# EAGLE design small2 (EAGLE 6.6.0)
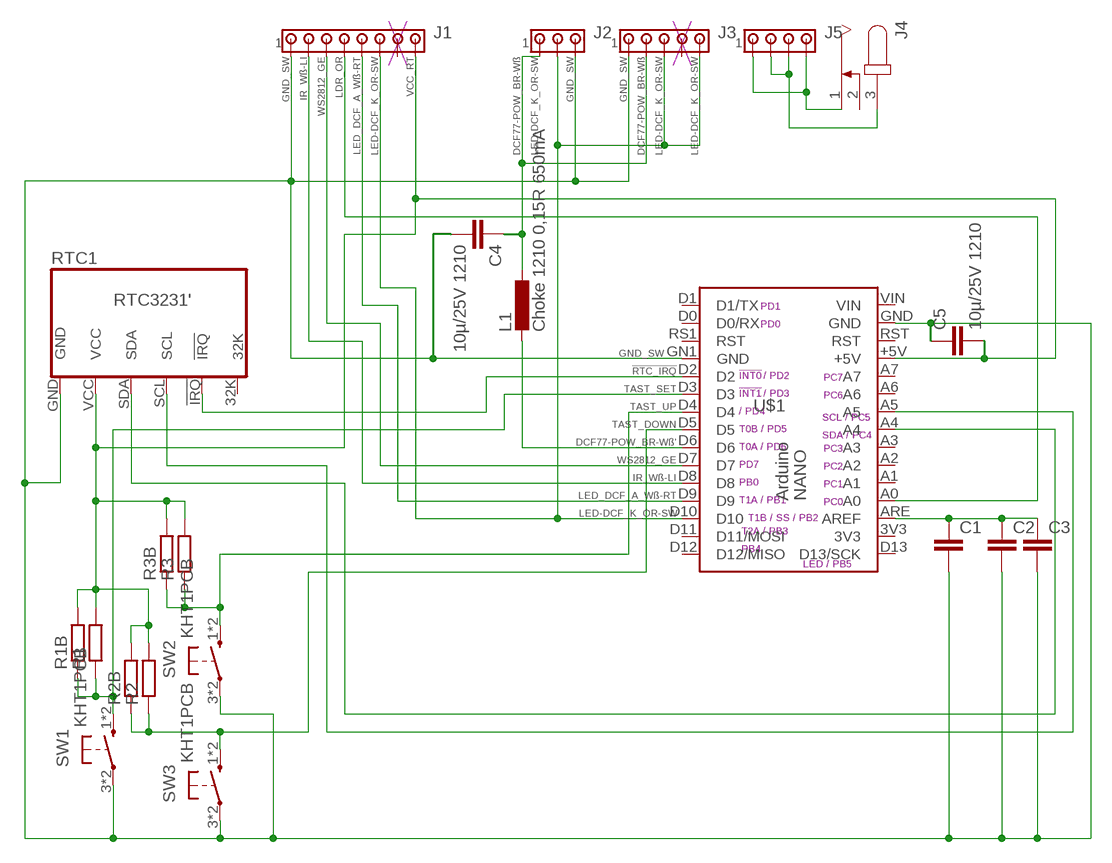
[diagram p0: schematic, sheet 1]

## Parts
C1  C-EU025-024X044  [C025-024X044]
C2  C-EU050-024X044  [C050-024X044]
C3  C-EUC0805  [C0805]
C4  10µ/25V 1210  C-EUC1210  [C1210]
C5  10µ/25V 1210  C-EUC1210  [C1210]
J1  MTA08-100  [10X08MTA]
J2  MTA03-100  [10X03MTA]
J3  MTA05-100  [10X05MTA]
J4  JACK-PLUG0  [SPC4077]
J5  MTA04-100  [10X04MTA]
L1  Choke 1210 0,15R 650mA  L-EUL2825P  [L2825P]
R1  R-EU_0204/5  [0204/5]
R1B  R-EU_M0805  [M0805]
R2  R-EU_0204/5  [0204/5]
R2B  R-EU_R0805  [R0805]
R3  R-EU_0204/5  [0204/5]
R3B  R-EU_M0805  [M0805]
RTC1  RTC3231'  [RTC3231"]
SW1  KHT1PCB  [OMRON_SWITCH]
SW2  KHT1PCB  [OMRON_SWITCH]
SW3  KHT1PCB  [OMRON_SWITCH]
U$1  ARDUINO_NANO3"  [ARDUINO_NANO3"]

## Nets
!RTC_IRQ: RTC1.!IRQ U$1.D2
DCF77-POW_BR-Wß: C4.1 J2.1 J3.2 L1.1
DCF77-POW_BR-Wß': L1.2 U$1.D6
GND_SW: C1.2 C2.2 C3.2 C4.2 C5.1 J1.1 J2.3 J3.1 RTC1.GND SW1.3(S) SW1.4(S) SW2.3(S) SW2.4(S) SW3.3(S) SW3.4(S) U$1.GN1(GND) U$1.GND
IR_Wß-LI: J1.2 U$1.D8
LDR_OR: J1.4 U$1.A0
LED-DCF_K_OR-SW: J1.6 J2.2 J3.3 J3.5 U$1.D10
LED_DCF_A_Wß-RT: J1.5 U$1.D9
N$2: RTC1.SDA U$1.A4
N$3: RTC1.SCL U$1.A5
N$6: C1.1 C2.1 C3.1 U$1.ARE(AREF)
N$78: J4.3 J5.2 J5.3
N$79: J4.1 J5.1 J5.4
TAST_DOWN: R2.1 R2B.1 SW3.1(P) SW3.2(P) U$1.D5
TAST_SET: R1.1 R1B.1 SW1.1(P) SW1.2(P) U$1.D3
TAST_UP: R3.1 R3B.1 SW2.1(P) SW2.2(P) U$1.D4
VCC_RT: C5.2 J1.8 R1.2 R1B.2 R2.2 R2B.2 R3.2 R3B.2 RTC1.VCC U$1.+5V
WS2812_GE: J1.3 U$1.D7
Unconnected: J1.7 J3.4 J4.2 RTC1.32K U$1.A1 U$1.A2 U$1.A3 U$1.A6 U$1.A7 U$1.D0(D0/RX) U$1.D1(D1/TX) U$1.D11(D11/MOSI) U$1.D12(D12/MISO) U$1.D13(D13/SCK) U$1.RS1(RST) U$1.RST

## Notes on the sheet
- GND_SW

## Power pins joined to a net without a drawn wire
3V3: U$1.3V3
VIN: U$1.VIN

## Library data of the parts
C1-C5 = rcl:C-EU: CAPACITOR, European symbol
J1 = con-amp:MTA08-100: AMP connector
J2 = con-amp:MTA03-100: AMP connector
J3 = con-amp:MTA05-100: AMP connector
J4 = con-jack:JACK-PLUG: DC POWER JACK Power Jack, DC, Right Angle, Through Hole, Rated 5A at 16VDC, PC Terminals Distributor: Farnell (www.Farnell.de) Drawing: 84N1161.pdf / 84N1162.pdf Manufacturer: SPC Technology (www.spctechnology.com) Type: SPC4077 / SPC 4078; OC_FARNELL: unknown; OC_NEWARK: unknown
J5 = con-amp:MTA04-100: AMP connector
L1 = rcl:L-EU: INDUCTOR, European symbol
R1 R1B R2 R2B R3 R3B = rcl:R-EU_: RESISTOR, European symbol
RTC1 = 1_____my_____1:RTC3231
SW1-SW3 = 1_____my_____1:KHT1
U$1 = 1_____my_____1:ARDUINO_NANO3

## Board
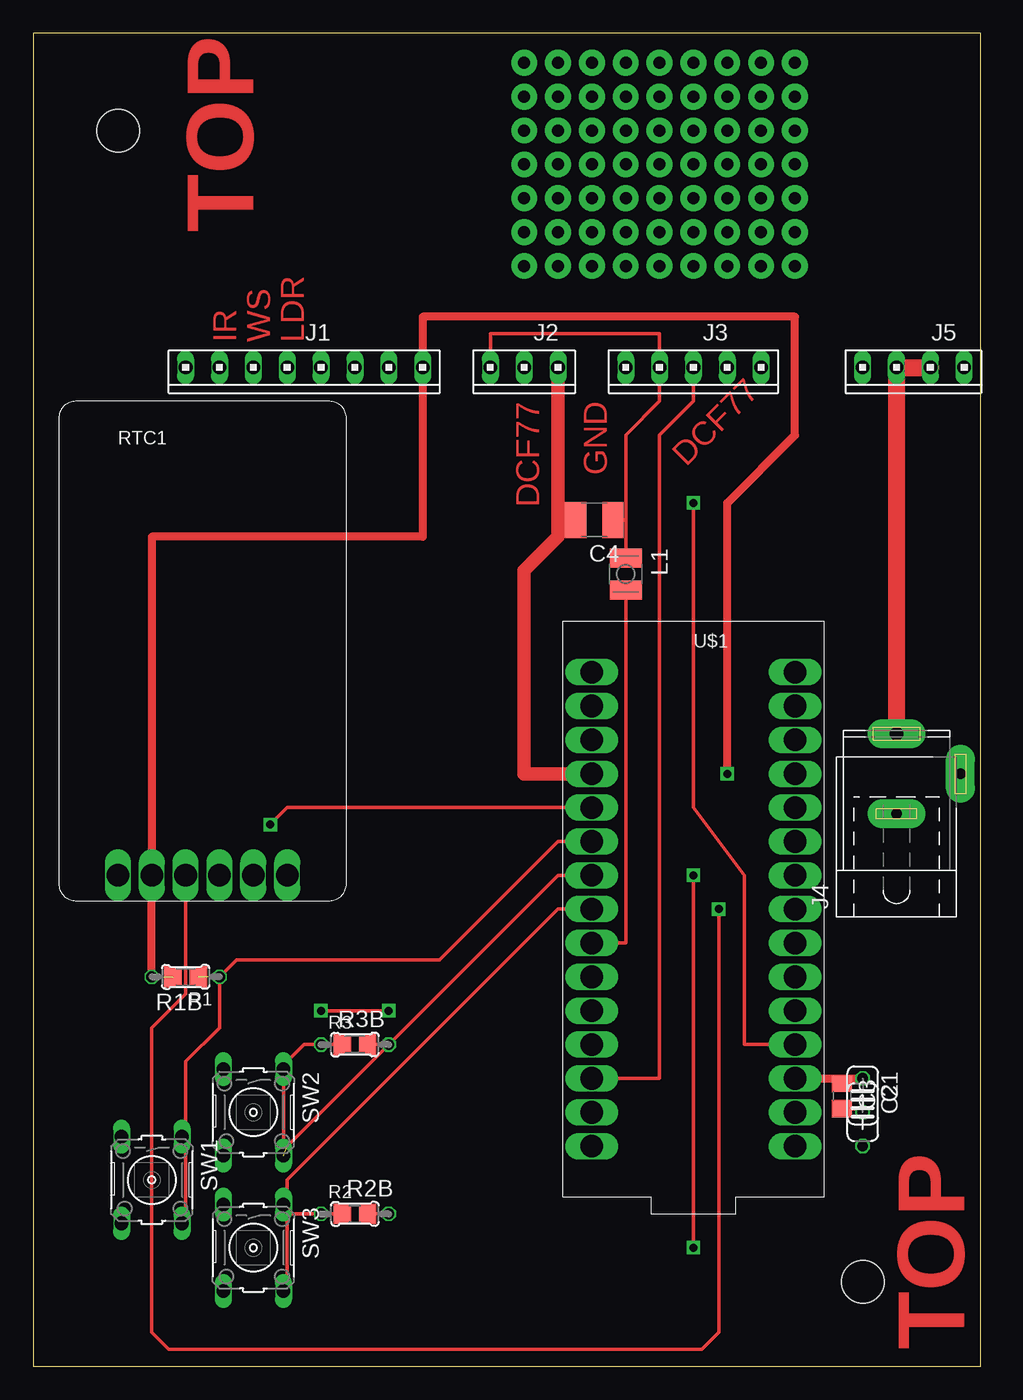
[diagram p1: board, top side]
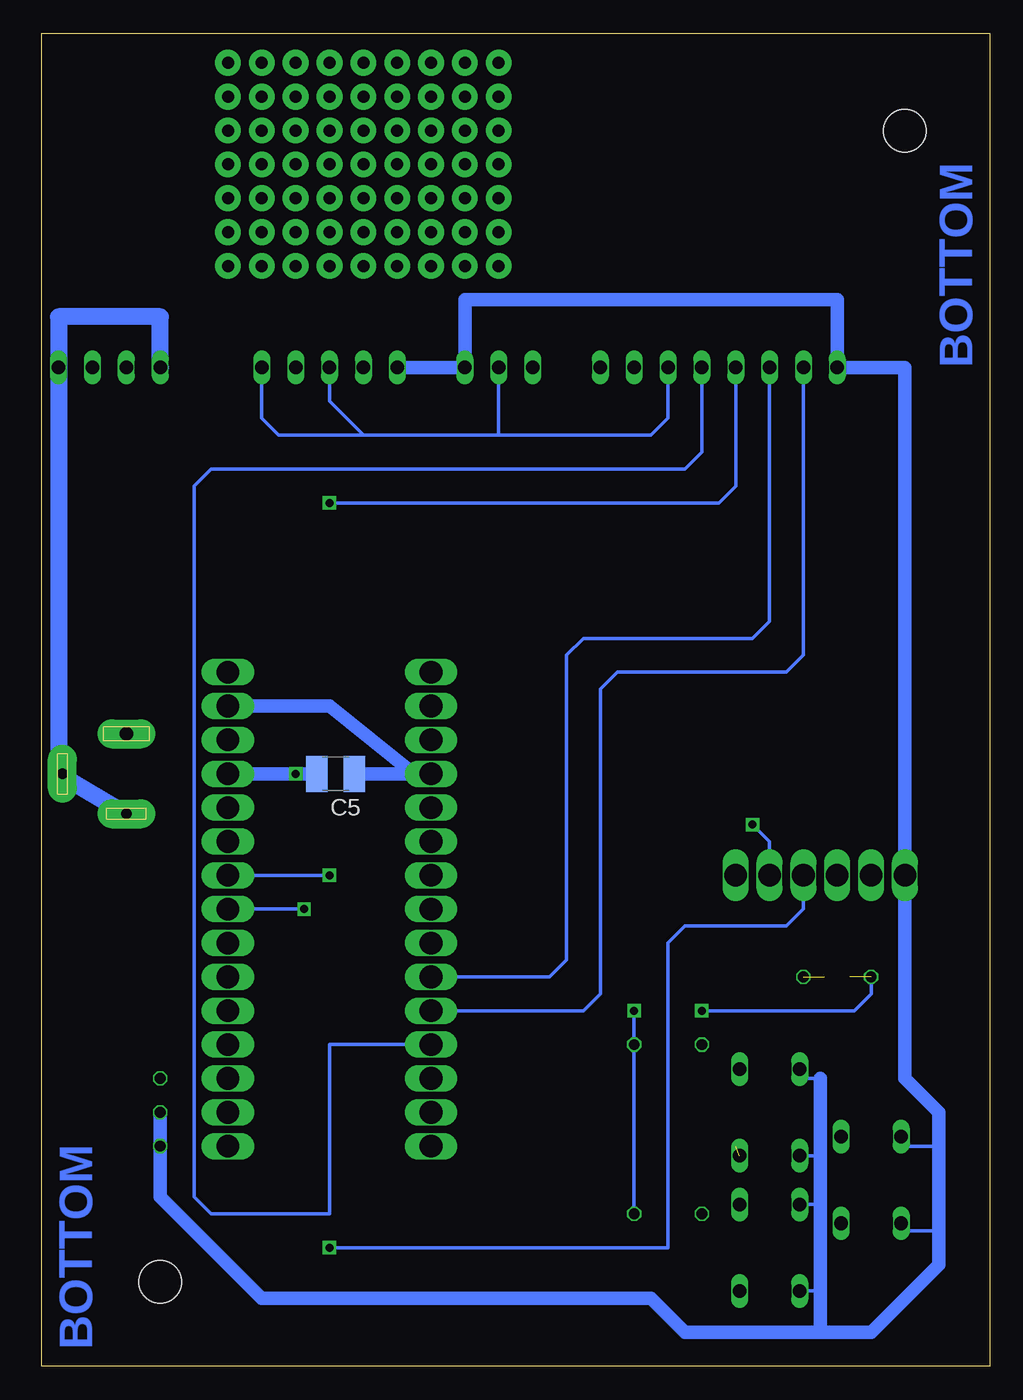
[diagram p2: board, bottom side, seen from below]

Size 71.11 x 100 mm. Coordinates in mm from the lower left corner, seen from the top.
Outline: 0,0 71.11,0 71.11,100 0,100 0,0
Copper layers (1*16): Top 0.035mm / dielectric 1.5mm / Bottom 0.035mm
Design rules "default *": minimum track width 10mil, minimum drill 24mil, track to track 8mil, track to pad 8mil, pad to pad 8mil, via to via 8mil, smd to smd 8mil, copper to edge 40mil, drill to drill 8mil, minimum pad ring 5mil, minimum via ring 8mil, stop-mask expansion 4mil, vias tented up to drill 0mil, thermal gap 10mil
Holes 3.2 mm at 6.35,92.71 62.23,6.35

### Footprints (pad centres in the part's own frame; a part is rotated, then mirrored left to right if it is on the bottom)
C025-024X044 = drill 0.813 octagon: 1 -1.27,0; 2 1.27,0
C050-024X044 = drill 0.813 octagon: 1 -2.54,0; 2 2.54,0
C0805 = smd 1.3 x 1.5: 1 -0.95,0; 2 0.95,0
C1210 = smd 1.6 x 2.7: 1 -1.4,0; 2 1.4,0
10X08MTA = drill 1.016 long: 1 8.89,0; 2 6.35,0; 3 3.81,0; 4 1.27,0; 5 -1.27,0; 6 -3.81,0; 7 -6.35,0; 8 -8.89,0
10X03MTA = drill 1.016 long: 1 2.54,0; 2 0,0; 3 -2.54,0
10X05MTA = drill 1.016 long: 1 5.08,0; 2 2.54,0; 3 0,0; 4 -2.54,0; 5 -5.08,0
SPC4077 = drill 0.8 pad 2.184 long: 1 -3,0; 2 0,-4.8 | drill 1 pad 2.184 long: 3 3,0
10X04MTA = drill 1.016 long: 1 3.81,0; 2 1.27,0; 3 -1.27,0; 4 -3.81,0
L2825P = smd 1.4 x 2.4: 1 -1.2,0; 2 1.2,0
0204/5 = drill 0.813 octagon: 1 -2.54,0; 2 2.54,0
M0805 = smd 1.3 x 1.6: 1 -0.95,0; 2 0.95,0
R0805 = smd 1.3 x 1.5: 1 -0.95,0; 2 0.95,0
RTC3231" = drill 1.7 pad 1.778 long: 32K 12.7,0; !IRQ 10.16,0; GND 0,0; SCL 7.62,0; SDA 5.08,0; VCC 2.54,0
OMRON_SWITCH = drill 1.016 long: 1 -3.251,2.261; 2 3.251,2.261; 3 -3.251,-2.261; 4 3.251,-2.261
ARDUINO_NANO3" = drill 1.7 pad 1.981 long: 3V3 15.24,-33.02; +5V 15.24,-7.62; A0 15.24,-27.94; A1 15.24,-25.4; A2 15.24,-22.86; A3 15.24,-20.32; A4 15.24,-17.78; A5 15.24,-15.24; A6 15.24,-12.7; A7 15.24,-10.16; ARE 15.24,-30.48; D0 0,-2.54; D1 0,0; D2 0,-10.16; D3 0,-12.7; D4 0,-15.24; D5 0,-17.78; D6 0,-20.32; D7 0,-22.86; D8 0,-25.4; D9 0,-27.94; D10 0,-30.48; D11 0,-33.02; D12 0,-35.56; D13 15.24,-35.56; GN1 0,-7.62; GND 15.24,-2.54; RS1 0,-5.08; RST 15.24,-5.08; VIN 15.24,0

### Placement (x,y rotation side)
C1  62.23,20.32 270 top
C2  62.23,19.05 270 top
C3  60.68,20.27 270 top
C4  42.09,63.5 180 top
C5  49.07,44.45 180 bottom
J1  20.32,74.93 180 top
J2  36.83,74.93 180 top
J3  49.53,74.93 180 top
J4  64.77,44.45 90 top
J5  66.04,74.93 180 top
L1  44.45,59.44 270 top
R1  11.43,29.21 180 top
R1B  11.43,29.21 180 top
R2  24.13,11.43 0 top
R2B  24.13,11.43 0 top
R3  24.13,24.13 0 top
R3B  24.13,24.13 0 top
RTC1  6.35,36.83 0 top
SW1  8.89,13.97 270 top
SW2  16.51,19.05 270 top
SW3  16.51,8.89 270 top
U$1  41.91,52.07 0 top

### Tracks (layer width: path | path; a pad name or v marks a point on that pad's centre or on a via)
!RTC_IRQ  (via drill 0.6)
  Top 0.254: U$1.D2 19.05,41.91 v17.78,40.64
  Bottom 0.254: v17.78,40.64 16.51,39.37 RTC1.!IRQ
DCF77-POW_BR-Wß
  Top 0.254: J2.1 34.29,77.47 46.99,77.47 J3.2 46.99,72.39 44.45,69.85 44.45,63.5 | 44.45,62.23 L1.1 44.45,63.5 | 44.45,63.5 C4.1
DCF77-POW_BR-Wß'
  Top 0.254: L1.2 44.45,31.75 U$1.D6
GND_SW
  Top 0.254: C4.2 39.37,63.5 | C3.2 62.23,19.32 C1.2
  Top 1.016: U$1.GN1 36.83,44.45 36.83,59.69 39.37,62.23 39.37,63.5 J2.3
  Bottom 0.254: SW1.4 6.35,10.16 3.81,10.16 | SW2.3 14.25,21.59 12.7,21.59 | 3.81,16.51 6.63,16.51 SW1.3 | SW2.4 12.7,15.8 12.7,16.51 | SW3.3 12.7,12.14 12.7,11.43 | SW3.4 12.7,5.64 12.7,6.35
  Bottom 0.61: C1.2 C2.2
  Bottom 1.016: 12.7,21.59 12.7,16.51 12.7,11.43 12.7,6.35 12.7,2.54 | 12.7,2.54 8.89,2.54 3.81,7.62 3.81,10.16 3.81,16.51 3.81,19.05 6.35,21.59 RTC1.GND 6.35,74.93 J1.1 11.43,80.01 39.37,80.01 J2.3 J3.1 | U$1.GND 49.53,49.53 43.18,44.45 U$1.GN1 C5.1 | C1.2 62.23,12.7 54.61,5.08 25.4,5.08 22.86,2.54 12.7,2.54
IR_Wß-LI
  Bottom 0.254: J1.2 13.97,53.34 15.24,52.07 27.94,52.07 29.21,50.8 29.21,27.94 30.48,26.67 U$1.D8
LDR_OR  (via drill 0.6)
  Top 0.254: v49.53,64.77 49.53,41.91 53.34,36.83 53.34,24.13 U$1.A0
  Bottom 0.254: J1.4 19.05,66.04 20.32,64.77 v49.53,64.77
LED-DCF_K_OR-SW
  Top 0.254: U$1.D10 46.99,21.59 46.99,69.85 49.53,72.39 J3.3
  Bottom 0.254: J1.6 24.13,71.12 25.4,69.85 36.83,69.85 | J2.2 36.83,69.85 | 46.99,69.85 49.53,72.39 J3.3 | 36.83,69.85 46.99,69.85 | J3.5 54.61,71.12 53.34,69.85 46.99,69.85
LED_DCF_A_Wß-RT
  Bottom 0.254: J1.5 21.59,68.58 22.86,67.31 58.42,67.31 59.69,66.04 59.69,12.7 58.42,11.43 49.53,11.43 49.53,24.13 U$1.D9
N$1  (via drill 0.9 pad 1.93)
  other vias: 41.91,82.55
N$2  (via drill 0.6)
  Top 0.254: RTC1.SDA 11.43,27.94 8.89,25.4 8.89,2.54 10.16,1.27 50.17,1.27 51.44,2.54 v51.44,34.29
  Bottom 0.254: U$1.A4 v51.44,34.29
N$3  (via drill 0.6)
  Top 0.254: v49.53,36.83 v49.53,8.89
  Bottom 0.254: RTC1.SCL 13.97,34.29 15.24,33.02 22.86,33.02 24.13,31.75 24.13,8.89 v49.53,8.89 | U$1.A5 v49.53,36.83
N$4  (via drill 0.9 pad 1.93)
  other vias: 44.45,82.55
N$5  (via drill 0.9 pad 1.93)
  other vias: 46.99,82.55
N$6
  Top 0.254: C2.1 60.68,21.59 C3.1
  Top 0.61: U$1.ARE C2.1
N$7  (via drill 0.9 pad 1.93)
  other vias: 46.99,85.09
N$8  (via drill 0.9 pad 1.93)
  other vias: 44.45,85.09
N$13  (via drill 0.9 pad 1.93)
  other vias: 41.91,85.09
N$14  (via drill 0.9 pad 1.93)
  other vias: 41.91,87.63
N$15  (via drill 0.9 pad 1.93)
  other vias: 44.45,87.63
N$16  (via drill 0.9 pad 1.93)
  other vias: 46.99,87.63
N$17  (via drill 0.9 pad 1.93)
  other vias: 49.53,87.63
N$18  (via drill 0.9 pad 1.93)
  other vias: 49.53,85.09
N$19  (via drill 0.9 pad 1.93)
  other vias: 49.53,82.55
N$20  (via drill 0.9 pad 1.93)
  other vias: 41.91,90.17
N$21  (via drill 0.9 pad 1.93)
  other vias: 44.45,90.17
N$22  (via drill 0.9 pad 1.93)
  other vias: 46.99,90.17
N$23  (via drill 0.9 pad 1.93)
  other vias: 49.53,90.17
N$24  (via drill 0.9 pad 1.93)
  other vias: 49.53,92.71
N$25  (via drill 0.9 pad 1.93)
  other vias: 46.99,92.71
N$26  (via drill 0.9 pad 1.93)
  other vias: 44.45,92.71
N$27  (via drill 0.9 pad 1.93)
  other vias: 41.91,92.71
N$28  (via drill 0.9 pad 1.93)
  other vias: 52.07,92.71
N$29  (via drill 0.9 pad 1.93)
  other vias: 52.07,90.17
N$30  (via drill 0.9 pad 1.93)
  other vias: 52.07,87.63
N$31  (via drill 0.9 pad 1.93)
  other vias: 52.07,85.09
N$32  (via drill 0.9 pad 1.93)
  other vias: 52.07,82.55
N$33  (via drill 0.9 pad 1.93)
  other vias: 39.37,82.55
N$34  (via drill 0.9 pad 1.93)
  other vias: 39.37,85.09
N$35  (via drill 0.9 pad 1.93)
  other vias: 39.37,87.63
N$36  (via drill 0.9 pad 1.93)
  other vias: 39.37,90.17
N$37  (via drill 0.9 pad 1.93)
  other vias: 39.37,92.71
N$38  (via drill 0.9 pad 1.93)
  other vias: 54.61,92.71
N$39  (via drill 0.9 pad 1.93)
  other vias: 54.61,90.17
N$40  (via drill 0.9 pad 1.93)
  other vias: 54.61,87.63
N$41  (via drill 0.9 pad 1.93)
  other vias: 54.61,85.09
N$42  (via drill 0.9 pad 1.93)
  other vias: 54.61,82.55
N$43  (via drill 0.9 pad 1.93)
  other vias: 36.83,82.55
N$44  (via drill 0.9 pad 1.93)
  other vias: 36.83,85.09
N$45  (via drill 0.9 pad 1.93)
  other vias: 36.83,87.63
N$46  (via drill 0.9 pad 1.93)
  other vias: 36.83,90.17
N$47  (via drill 0.9 pad 1.93)
  other vias: 36.83,92.71
N$48  (via drill 0.9 pad 1.93)
  other vias: 36.83,95.25
N$49  (via drill 0.9 pad 1.93)
  other vias: 39.37,95.25
N$50  (via drill 0.9 pad 1.93)
  other vias: 41.91,95.25
N$51  (via drill 0.9 pad 1.93)
  other vias: 44.45,95.25
N$52  (via drill 0.9 pad 1.93)
  other vias: 46.99,95.25
N$53  (via drill 0.9 pad 1.93)
  other vias: 49.53,95.25
N$54  (via drill 0.9 pad 1.93)
  other vias: 52.07,95.25
N$55  (via drill 0.9 pad 1.93)
  other vias: 54.61,95.25
N$56  (via drill 0.9 pad 1.93)
  other vias: 54.61,97.79
N$57  (via drill 0.9 pad 1.93)
  other vias: 52.07,97.79
N$58  (via drill 0.9 pad 1.93)
  other vias: 49.53,97.79
N$59  (via drill 0.9 pad 1.93)
  other vias: 46.99,97.79
N$60  (via drill 0.9 pad 1.93)
  other vias: 44.45,97.79
N$61  (via drill 0.9 pad 1.93)
  other vias: 41.91,97.79
N$62  (via drill 0.9 pad 1.93)
  other vias: 39.37,97.79
N$63  (via drill 0.9 pad 1.93)
  other vias: 36.83,97.79
N$64  (via drill 0.9 pad 1.93)
  other vias: 57.15,97.79
N$65  (via drill 0.9 pad 1.93)
  other vias: 57.15,95.25
N$66  (via drill 0.9 pad 1.93)
  other vias: 57.15,92.71
N$67  (via drill 0.9 pad 1.93)
  other vias: 57.15,90.17
N$68  (via drill 0.9 pad 1.93)
  other vias: 57.15,87.63
N$69  (via drill 0.9 pad 1.93)
  other vias: 57.15,85.09
N$70  (via drill 0.9 pad 1.93)
  other vias: 57.15,82.55
N$78
  Top 1.27: J5.3 J5.2 J4.3
N$79
  Bottom 1.27: J5.1 62.23,78.74 69.85,78.74 J5.4 69.85,44.45 J4.1
TAST_DOWN
  Top 0.254: 19.05,13.97 39.37,34.29 U$1.D5 | 19.05,11.43 19.05,6.35 SW3.2 | 19.05,13.97 19.05,11.43 | 19.05,11.43 19.05,12.14 SW3.1 | 19.05,11.43 R2.1 R2B.1 | 19.05,11.43 19.05,13.97
TAST_SET  (1 unrouted)
  Top 0.254: U$1.D3 39.37,39.37 30.48,30.48 15.24,30.48 R1.1 13.97,25.4 11.43,22.86 11.43,16.51 | 11.43,16.51 11.43,11.43 SW1.2 | 11.43,16.51 SW1.1
TAST_UP  (1 unrouted)
  Top 0.254: 19.05,16.51 39.37,36.83 U$1.D4 | SW2.2 SW2.1 19.05,21.59 19.05,22.86 20.32,24.13 R3.1 R3B.1
VCC_RT  (via drill 0.6)  (1 unrouted)
  Top 0.254: v21.59,26.67 v26.67,26.67 | R2B.2 R2.2 | R3B.2 R3.2
  Top 0.61: v52.07,44.45 52.07,64.77 57.15,69.85 57.15,78.74 29.21,78.74 J1.8 29.21,62.23 8.89,62.23 RTC1.VCC R1.2
  Bottom 0.254: R2.2 R3.2 v26.67,26.67 | R1.2 8.89,27.94 10.16,26.67 v21.59,26.67
  Bottom 1.016: U$1.+5V v52.07,44.45 C5.2
WS2812_GE
  Bottom 0.254: J1.3 16.51,55.88 17.78,54.61 30.48,54.61 31.75,53.34 31.75,30.48 33.02,29.21 U$1.D7

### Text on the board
Top: TOP | IR | WS | LDR | DCF77 | DCF77 | GND | TOP
Bottom: BOTTOM | BOTTOM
